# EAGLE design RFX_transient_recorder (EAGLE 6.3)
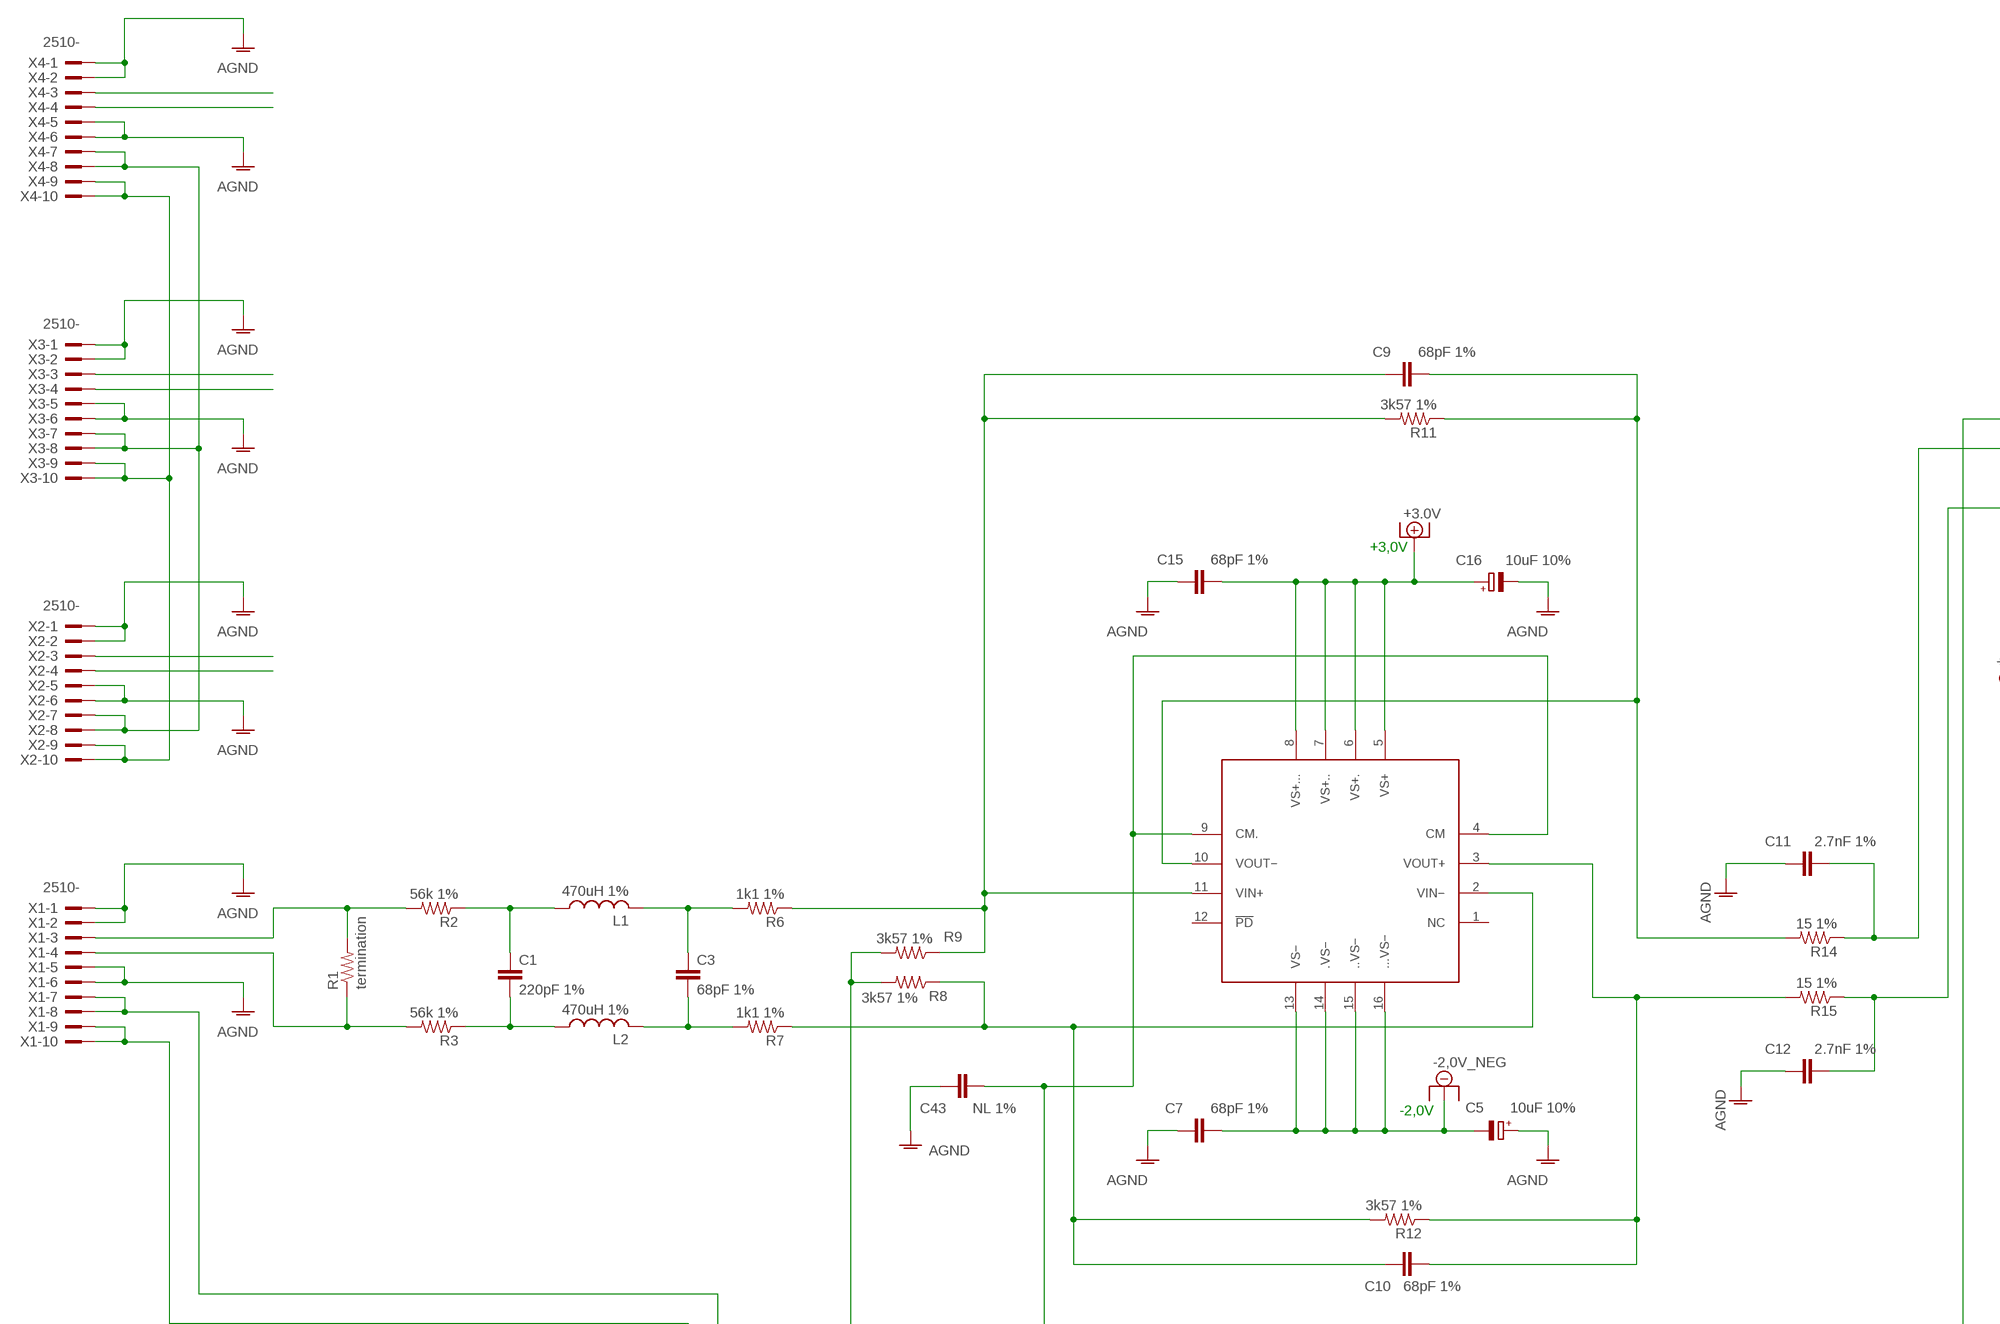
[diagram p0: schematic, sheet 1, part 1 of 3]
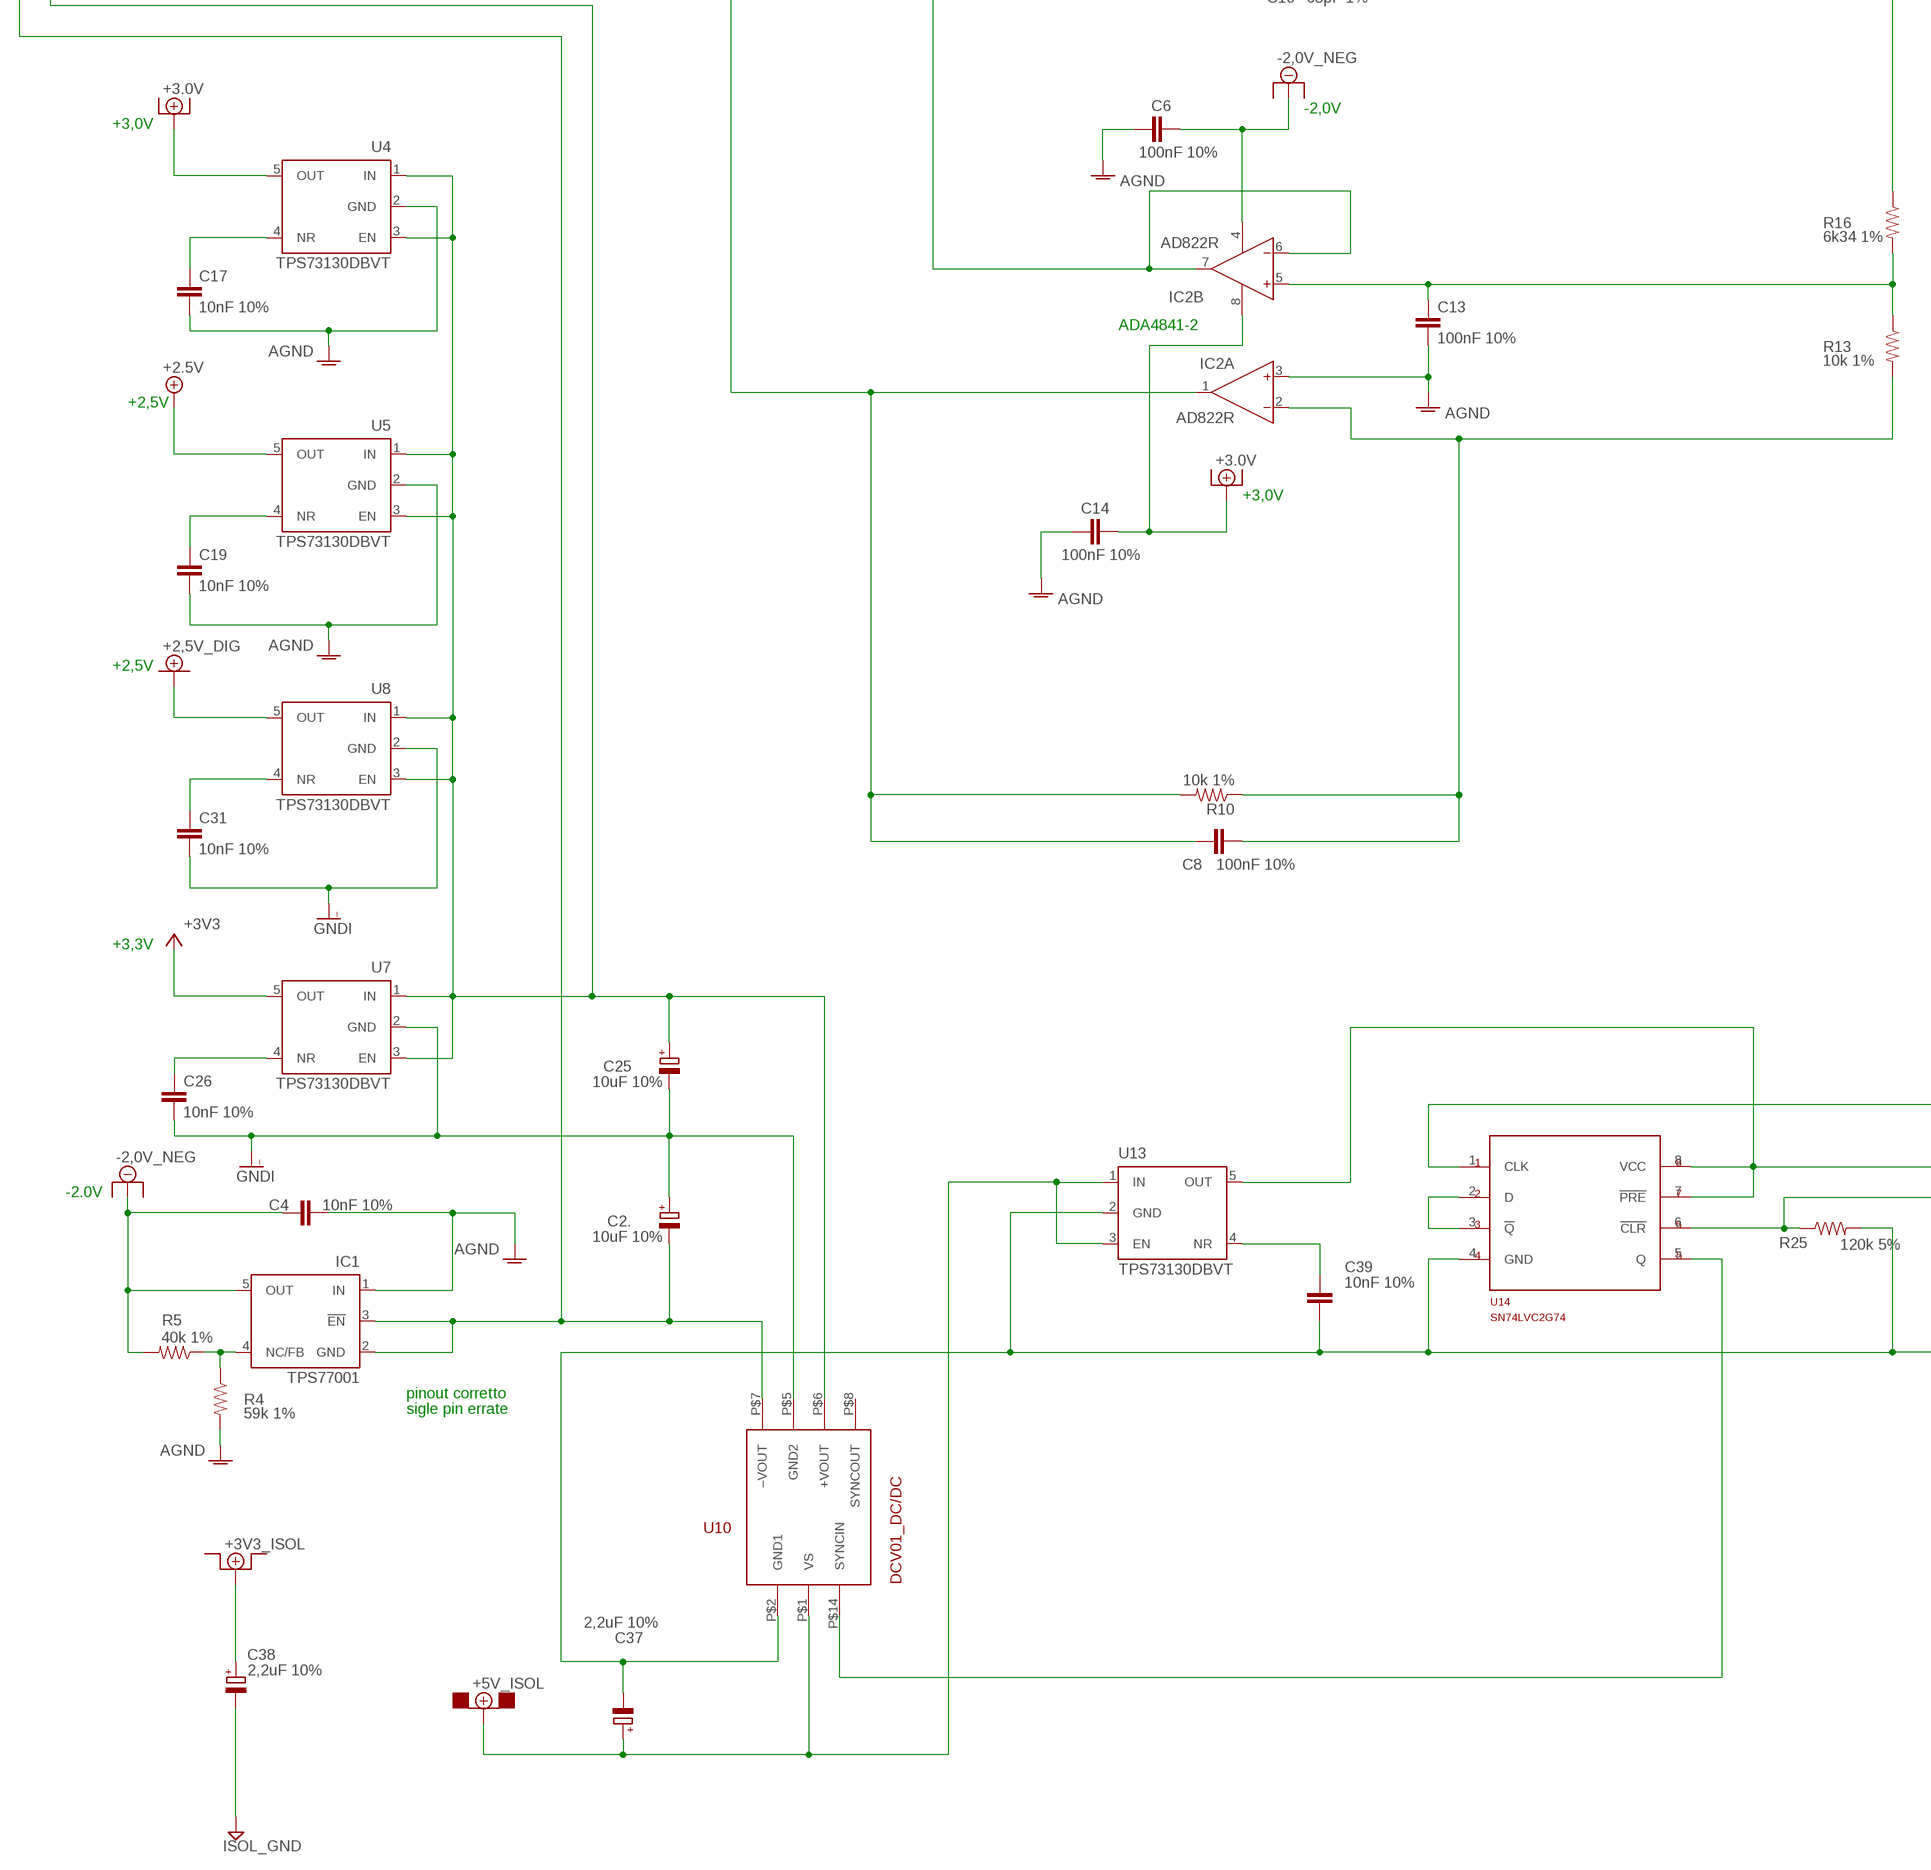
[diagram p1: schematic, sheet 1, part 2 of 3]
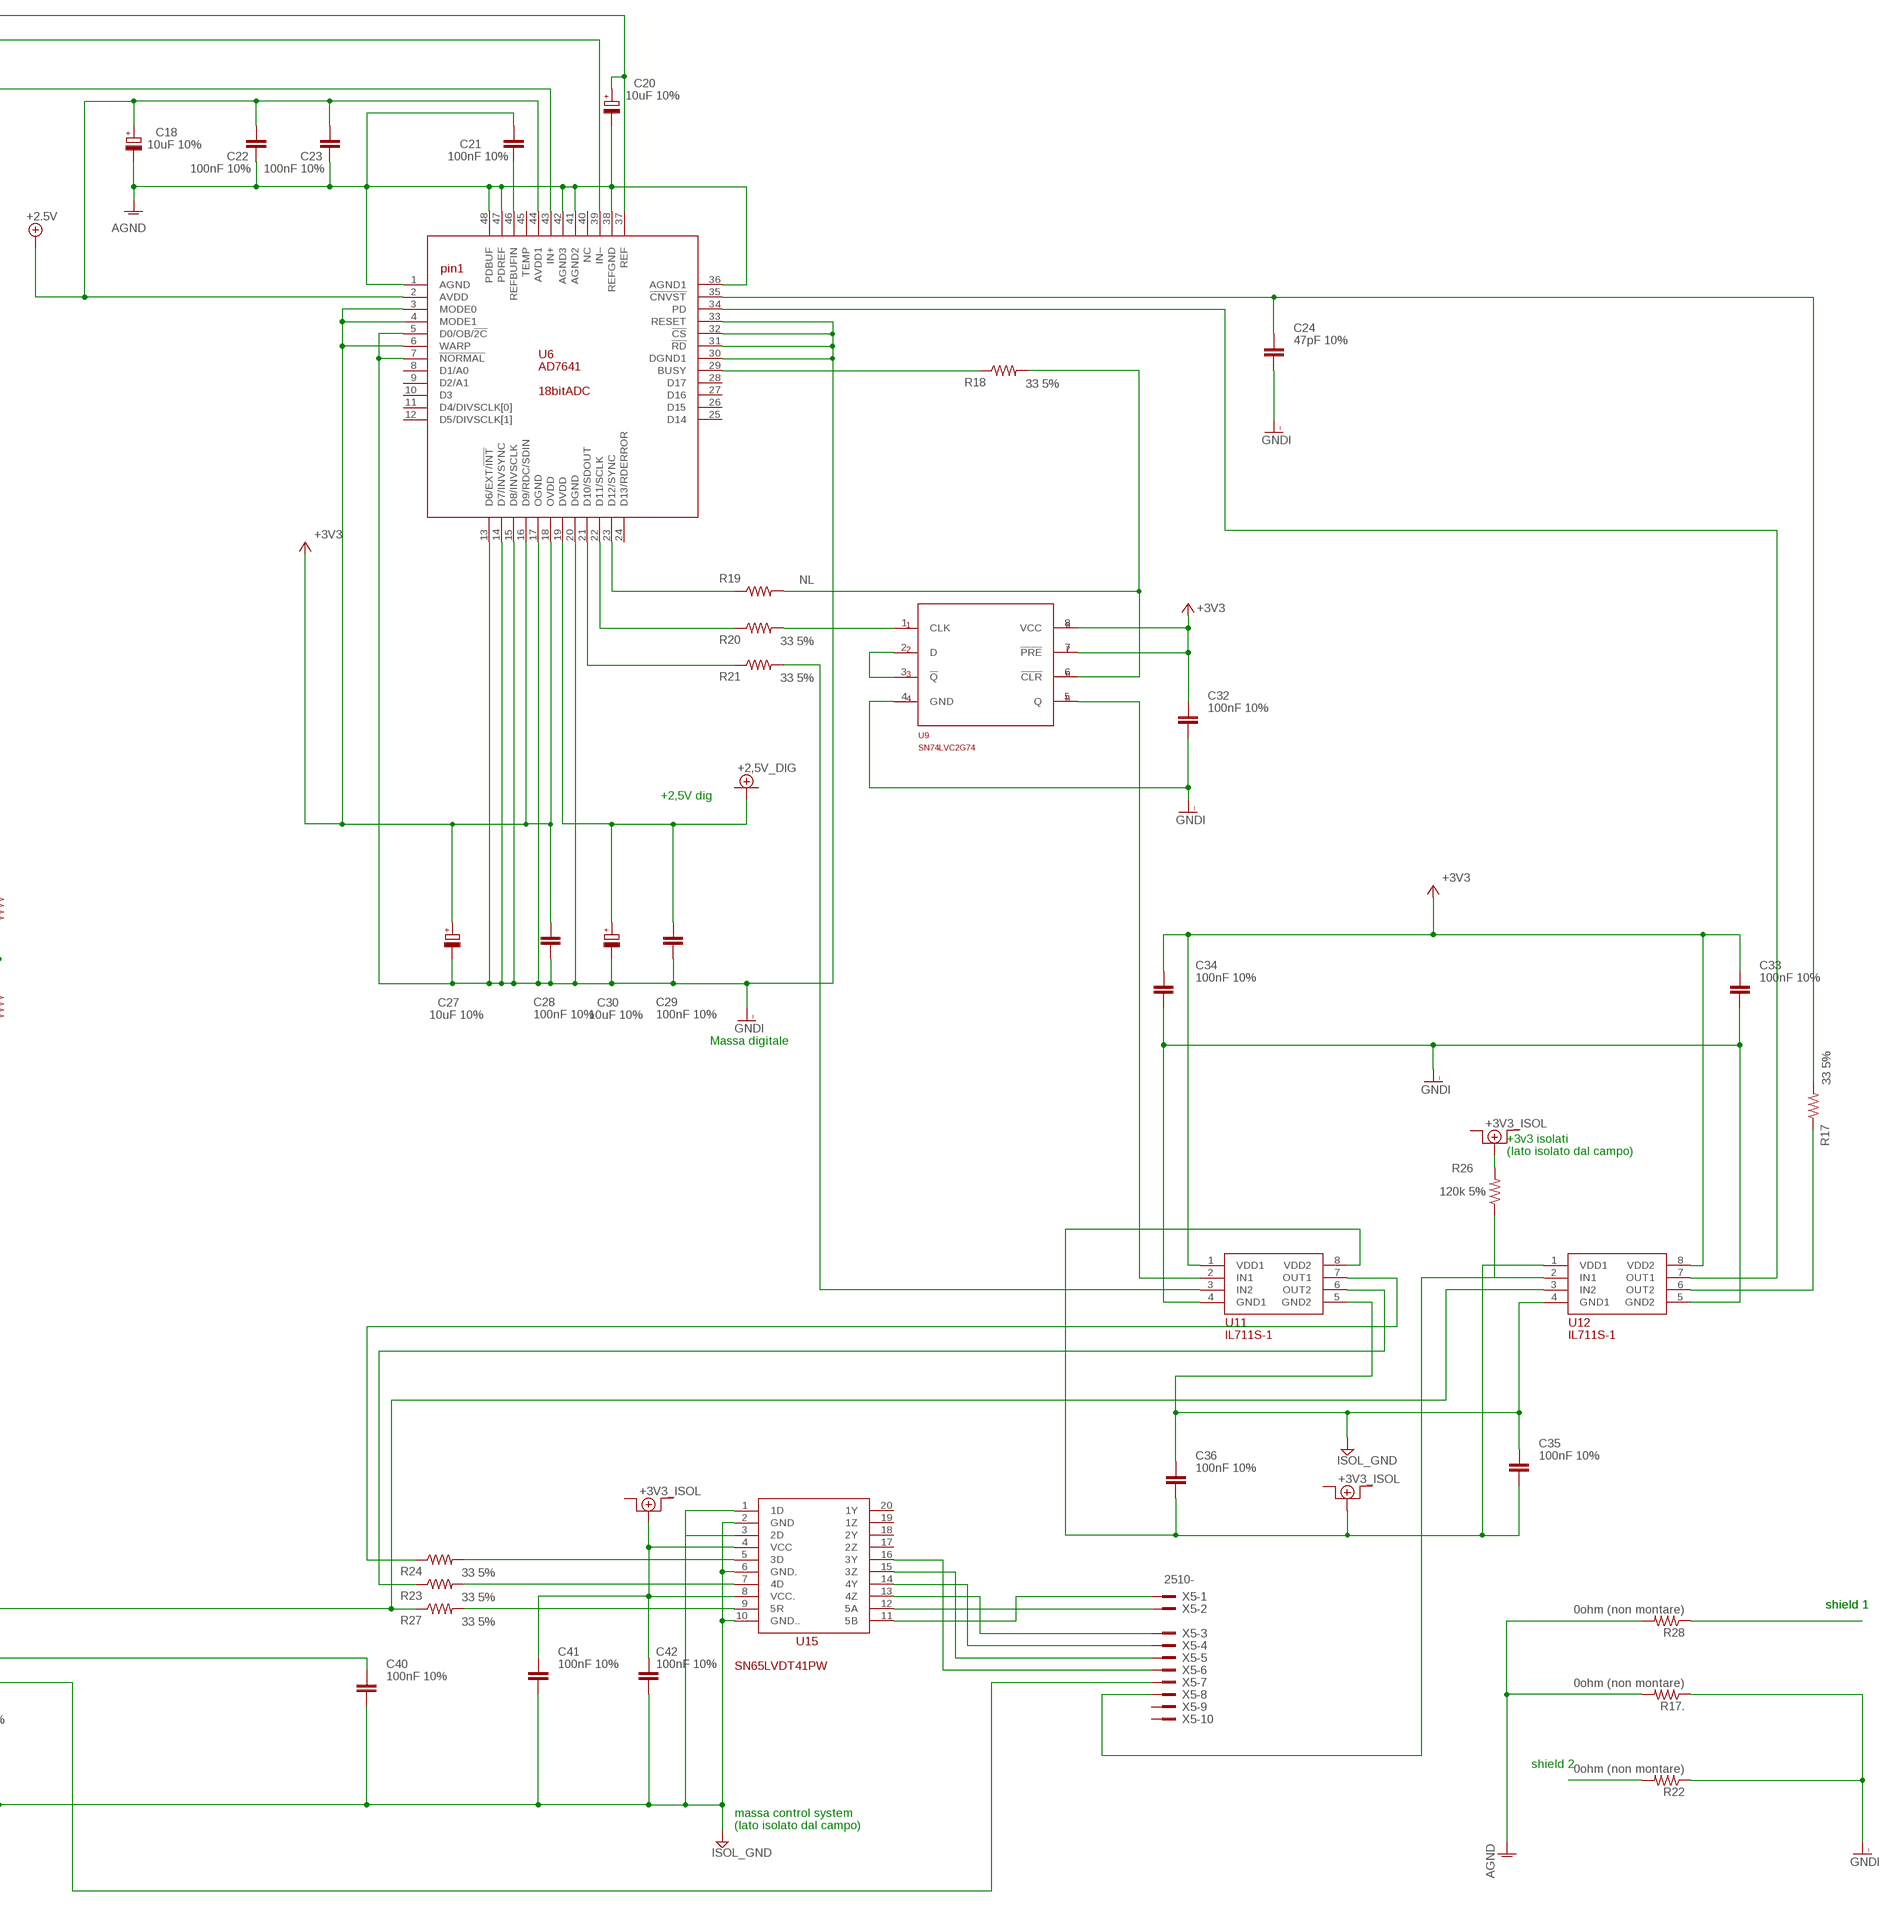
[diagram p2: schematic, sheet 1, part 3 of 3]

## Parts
C1  220pF 1%  C-EUC0402  [C0402]
C2.  10uF 10%  CPOL-EUSMCA  [SMC_A]
C3  68pF 1%  C-EUC0402  [C0402]
C4  10nF 10%  C-EUC0402  [C0402]
C5  10uF 10%  CPOL-EUSMCA  [SMC_A]
C6  100nF 10%  C-EUC0402  [C0402]
C7  68pF 1%  C-EUC0402  [C0402]
C8  100nF 10%  C-EUC0402  [C0402]
C9  68pF 1%  C-EUC0402  [C0402]
C10  68pF 1%  C-EUC0402  [C0402]
C11  2.7nF 1%  C-EUC0402  [C0402]
C12  2.7nF 1%  C-EUC0402  [C0402]
C13  100nF 10%  C-EUC0402  [C0402]
C14  100nF 10%  C-EUC0402  [C0402]
C15  68pF 1%  C-EUC0402  [C0402]
C16  10uF 10%  CPOL-EUSMCA  [SMC_A]
C17  10nF 10%  C-EUC0402  [C0402]
C18  10uF 10%  CPOL-EUSMCA  [SMC_A]
C19  10nF 10%  C-EUC0402  [C0402]
C20  10uF 10%  CPOL-EUSMCA  [SMC_A]
C21  100nF 10%  C-EUC0402  [C0402]
C22  100nF 10%  C-EUC0402  [C0402]
C23  100nF 10%  C-EUC0402  [C0402]
C24  47pF 10%  C-EUC0402  [C0402]
C25  10uF 10%  CPOL-EUSMCA  [SMC_A]
C26  10nF 10%  C-EUC0402  [C0402]
C27  10uF 10%  CPOL-EUSMCA  [SMC_A]
C28  100nF 10%  C-EUC0402  [C0402]
C29  100nF 10%  C-EUC0402  [C0402]
C30  10uF 10%  CPOL-EUSMCA  [SMC_A]
C31  10nF 10%  C-EUC0402  [C0402]
C32  100nF 10%  C-EUC0402  [C0402]
C33  100nF 10%  C-EUC0402  [C0402]
C34  100nF 10%  C-EUC0402  [C0402]
C35  100nF 10%  C-EUC0402  [C0402]
C36  100nF 10%  C-EUC0402  [C0402]
C37  2,2uF 10%  CPOL-EUSMCA  [SMC_A]
C38  2,2uF 10%  CPOL-EUSMCA  [SMC_A]
C39  10nF 10%  C-EUC0402  [C0402]
C40  100nF 10%  C-EUC0402  [C0402]
C41  100nF 10%  C-EUC0402  [C0402]
C42  100nF 10%  C-EUC0402  [C0402]
C43  NL 1%  C-EUC0402  [C0402]
IC1  TPS77001  [SOT23-DBV]
IC2  AD822R  [SO8]
L1  470uH 1%  L-USL3216C  [L3216C]
L2  470uH 1%  L-USL3216C  [L3216C]
R1  termination  R-US_R0402  [R0402]
R2  56k 1%  R-US_R0402  [R0402]
R3  56k 1%  R-US_R0402  [R0402]
R4  59k 1%  R-US_R0402  [R0402]
R5  40k 1%  R-US_R0402  [R0402]
R6  1k1 1%  R-US_R0402  [R0402]
R7  1k1 1%  R-US_R0402  [R0402]
R8  3k57 1%  R-US_R0402  [R0402]
R9  3k57 1%  R-US_R0402  [R0402]
R10  10k 1%  R-US_R0402  [R0402]
R11  3k57 1%  R-US_R0402  [R0402]
R12  3k57 1%  R-US_R0402  [R0402]
R13  10k 1%  R-US_R0402  [R0402]
R14  15 1%  R-US_R0402  [R0402]
R15  15 1%  R-US_R0402  [R0402]
R16  6k34 1%  R-US_R0402  [R0402]
R17  33 5%  R-US_R0402  [R0402]
R17.  0ohm (non montare)  R-US_R0402  [R0402]
R18  33 5%  R-US_R0402  [R0402]
R19  NL  R-US_R0402  [R0402]
R20  33 5%  R-US_R0402  [R0402]
R21  33 5%  R-US_R0402  [R0402]
R22  0ohm (non montare)  R-US_R0402  [R0402]
R23  33 5%  R-US_R0402  [R0402]
R24  33 5%  R-US_R0402  [R0402]
R25  120k 5%  R-US_R0402  [R0402]
R26  120k 5%  R-US_R0402  [R0402]
R27  33 5%  R-US_R0402  [R0402]
R28  0ohm (non montare)  R-US_R0402  [R0402]
U4  TPS73130DBVT  [SOT23-DBV]
U5  TPS73130DBVT  [SOT23-DBV]
U6  AD7641  [QFP-7X7-48]
U7  TPS73130DBVT  [SOT23-DBV]
U8  TPS73130DBVT  [SOT23-DBV]
U9  SN74LVC2G74  [SO-08]
U10  DCV01_DC/DCDCV010505DP_DC/DC_CONVERTER  [DCV10_DC/DC]
U11  IL711S-1  [SO-08]
U12  IL711S-1  [SO-08]
U13  TPS73130DBVT  [SOT23-DBV]
U14  SN74LVC2G74  [SO-08]
U15  SN65LVDT41PW  [TSSOP16]
U$1  THS4520_QFN16  [QFN16]
X1  2510-  [PAK100/2500-10]
X2  2510-  [PAK100/2500-10]
X3  2510-  [PAK100/2500-10]
X4  2510-  [PAK100/2500-10]
X5  2510-  [PAK100/2500-10]

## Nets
+2.5V: C18.+ C22.2 C23.2 U5.5(OUT) U6.2(AVDD) U6.44(AVDD1)
+2.5V_DIG: C29.2 C30.+ U6.19(DVDD) U8.5(OUT) ; supply symbol labelled +2,5V_DIG
+3.0V: C14.2 C15.2 C16.+ IC2.8(P:V+) U4.5(OUT) U$1.5(VS+) U$1.6(VS+.) U$1.7(VS+..) U$1.8(VS+...)
+3V3: C27.+ C28.2 C32.2 C33.2 C34.2 U6.3(MODE0) U6.4(MODE1) U6.6(WARP) U6.16(D9/RDC/SDIN) U6.18(OVDD) U7.5(OUT) U9.7(!PRE!) U9.8(VCC) U11.1(VDD1) U12.8(VDD2)
+3V3_ISOL: C35.1 C36.1 C38.+ C41.2 C42.2 R26.2 U11.8(VDD2) U12.1(VDD1) U15.4(VCC) U15.8(VCC.)
+5V_ISOL: C37.+ U10.P$1(VS) U13.1(IN) U13.3(EN)
-2.0V_NEG: C4.1 C5.- C6.2 C7.2 IC1.5(OUT) IC2.4(P:V-) R5.2 U$1.13(VS−) U$1.14(.VS−) U$1.15(..VS−) U$1.16(...VS−) ; supply symbol labelled -2,0V_NEG
AGND: C4.2 C5.+ C6.1 C7.1 C11.1 C12.1 C13.2 C14.1 C15.1 C16.- C17.2 C18.- C19.2 C20.- C21.2 C22.1 C23.1 C43.1 IC1.1(IN) IC2.3(A:IN+) R4.2 R17..2 R28.2 U4.2(GND) U5.2(GND) U6.1(AGND) U6.36(AGND1) U6.38(REFGND) U6.41(AGND2) U6.42(AGND3) U6.47(PDREF) U6.48(PDBUF) X1.1 X1.2 X1.5 X1.6 X2.1 X2.2 X2.5 X2.6 X3.1 X3.2 X3.5 X3.6 X4.1 X4.2 X4.5 X4.6
GNDI: C2..+ C24.1 C25.- C26.2 C27.- C28.1 C29.1 C30.- C31.2 C32.1 C33.1 C34.1 R17..1 R22.1 U6.5(D0/OB/!2C!) U6.7(!NORMAL!) U6.13(D6/EXT/!INT!) U6.14(D7/INVSYNC) U6.15(D8/INVSCLK) U6.17(OGND) U6.20(DGND) U6.30(DGND1) U6.31(!RD!) U6.32(!CS!) U6.33(RESET) U7.2(GND) U8.2(GND) U9.4(GND) U10.P$5(GND2) U11.4(GND1) U12.5(GND2)
ISOL_GND: C35.2 C36.2 C37.- C38.- C39.1 C40.1 C41.1 C42.1 R25.2 U10.P$2(GND1) U11.5(GND2) U12.4(GND1) U13.2(GND) U14.4(GND) U15.1(1D) U15.2(GND) U15.3(2D) U15.6(GND.) U15.10(GND..)
N$1: C3.1 L1.2 R6.2
N$2: C1.1 L1.1 R2.1
N$3: C3.2 L2.2 R7.2
N$4: C1.2 L2.1 R3.1
N$5: C9.1 R6.1 R9.1 R11.2 U$1.11(VIN+)
N$6: C10.1 R7.1 R8.1 R12.2 U$1.2(VIN−)
N$7: R20.2 U9.1(CLK)
N$8: R1.2 R2.2 X1.3
N$9: R1.1 R3.2 X1.4
N$10: C9.2 R11.1 R14.2 U$1.10(VOUT−)
N$11: C10.2 R12.1 R15.2 U$1.3(VOUT+)
N$12: C11.2 R14.1 U6.39(IN–)
N$13: C12.2 R15.1 U6.43(IN+)
N$14: R28.1
N$15: R22.2
N$16: C2..- IC1.2(GND) IC1.3(!EN) U10.P$7(–VOUT) X1.9 X1.10
N$17: C17.1 U4.4(NR)
N$18: C25.+ U4.1(IN) U4.3(EN) U5.1(IN) U5.3(EN) U7.1(IN) U7.3(EN) U8.1(IN) U8.3(EN) U10.P$6(+VOUT) X1.7 X1.8
N$19: X2.3
N$20: C19.1 U5.4(NR)
N$21: X2.4
N$22: X2.9 X2.10 X3.9 X3.10 X4.9 X4.10
N$23: C31.1 U8.4(NR)
N$24: X2.7 X2.8 X3.7 X3.8 X4.7 X4.8
N$25: X3.3
N$26: C26.1 U7.4(NR)
N$27: IC1.4(NC/FB) R4.1 R5.1
N$28: C43.2 IC2.6(B:IN-) IC2.7(B:OUT) U$1.4(CM) U$1.9(CM.)
N$29: X3.4
N$30: C13.1 IC2.5(B:IN+) R13.1 R16.2
N$31: R20.1 U6.22(D11/SCLK)
N$32: C20.+ R16.1 U6.37(REF)
N$33: C21.1 U6.46(REFBUFIN)
N$34: U15.11(5B) X5.1
N$35: U15.12(5A) X5.2
N$36: R19.1 U6.23(D12/SYNC)
N$37: R18.2 R19.2 U9.6(!CLR!)
N$38: R18.1 U6.29(BUSY)
N$39: U9.2(D) U9.3(!Q!)
N$40: C8.1 IC2.1(A:OUT) R8.2 R9.2 R10.2
N$41: C8.2 IC2.2(A:IN-) R10.1 R13.2
N$42: U9.5(Q) U11.2(IN1)
N$43: R21.1 U6.21(D10/SDOUT)
N$44: R21.2 U11.3(IN2)
N$45: C24.2 R17.2 U6.35(!CNVST!)
N$46: R17.1 U12.6(OUT2)
N$47: U6.34(PD) U12.7(OUT1)
N$48: X4.3
N$49: X4.4
N$50: R27.1 U12.3(IN2) U14.1(CLK)
N$51: R24.2 U15.5(3D)
N$52: R23.2 U15.7(4D)
N$53: R24.1 U11.7(OUT1)
N$54: R23.1 U11.6(OUT2)
N$55: U15.13(4Z) X5.3
N$56: R27.2 U15.9(5R)
N$57: R26.1 U12.2(IN1) X5.8
N$58: U15.14(4Y) X5.4
N$59: U14.2(D) U14.3(!Q!)
N$60: R25.1 U14.6(!CLR!) X5.7
N$61: U10.P$14(SYNCIN) U14.5(Q)
N$62: C40.2 U13.5(OUT) U14.7(!PRE!) U14.8(VCC)
N$63: U15.15(3Z) X5.5
N$64: C39.2 U13.4(NR)
N$65: U15.16(3Y) X5.6
Unconnected: U6.8(D1/A0) U6.9(D2/A1) U6.10(D3) U6.11(D4/DIVSCLK[0]) U6.12(D5/DIVSCLK[1]) U6.24(D13/RDERROR) U6.25(D14) U6.26(D15) U6.27(D16) U6.28(D17) U6.40(NC) U6.45(TEMP) U10.P$8(SYNCOUT) U15.17(2Z) U15.18(2Y) U15.19(1Z) U15.20(1Y) U$1.1(NC) U$1.12(!PD!) X5.9 X5.10

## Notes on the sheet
- +3,0V
- -2,0V
- +2,5V dig
- -2,0V
- +3,0V
- ADA4841-2
- Massa digitale
- +2,5V
- +3,0V
- +3v3 isolati
- (lato isolato dal campo)
- +2,5V
- +3,3V
- shield 1 | shield 1
- -2.0V
- shield 2
- massa control system
- (lato isolato dal campo)
- pinout corretto
- sigle pin errate

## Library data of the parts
C1 C3 C4 C6-C15 C17 C19 C21-C24 C26 C28 C29 C31-C36 C39-C43 = resistor:C-EU: CAPACITOR, European symbol
C2. C5 C16 C18 C20 C25 C27 C30 C37 C38 = resistor:CPOL-EU: POLARIZED CAPACITOR, European symbol
IC1 = texas:TPS770*: ULTRALOW-POWER 50-mA LOW-DROPOUT LINEAR REGULATORS 50-mA Low-Dropout Regulator Source: http://focus.ti.com/lit/ds/symlink/tps77001.pdf; MF: TEXAS INSTRUMENTS; MPN: TPS77001DBVT; OC_FARNELL: 8461554; OC_NEWARK: 77C1171
IC2 = analog-devices:AD822: Single-Supply, Rail-to-Rail Low Power FET-Input Op Amp Source: http://www.analog.com/static/imported-files/data_sheets/AD822.pdf; MF: ANALOG DEVICES; MPN: AD822BRZ; OC_FARNELL: 1651303
L1 L2 = resistor:L-US: INDUCTOR, American symbol
R1-R17 R17. R18-R28 = resistor:R-US_: RESISTOR, American symbol
U4 U5 U7 U8 U13 = TPS73130DBVT:TPS73130DBVT
U6 = AD7641:AD7641
U9 U14 = SN74LVC2G74DCUR_SOP8:SN74LVC2G74
U10 = DCV01_DCDC:DCV01_DC/DC
U11 U12 = IL711S-1 SOIC8:IL711S-1
U15 = SN65LVDT41PW-TSSOP20:SN65LVDT41PW: MEMORY STICK™ INTERCONNECT EXTENDER CHIPSET WITH LVDS
U$1 = THS4520 QFN16:THS4520_QFN16
X1-X5 = con-3m:2510-: 3M (TM) Pak 100 4-Wall Header Source: 3M; MF: 3M; MPN: 2510-6002UB; OC_FARNELL: 9838244; OC_NEWARK: 46F4725

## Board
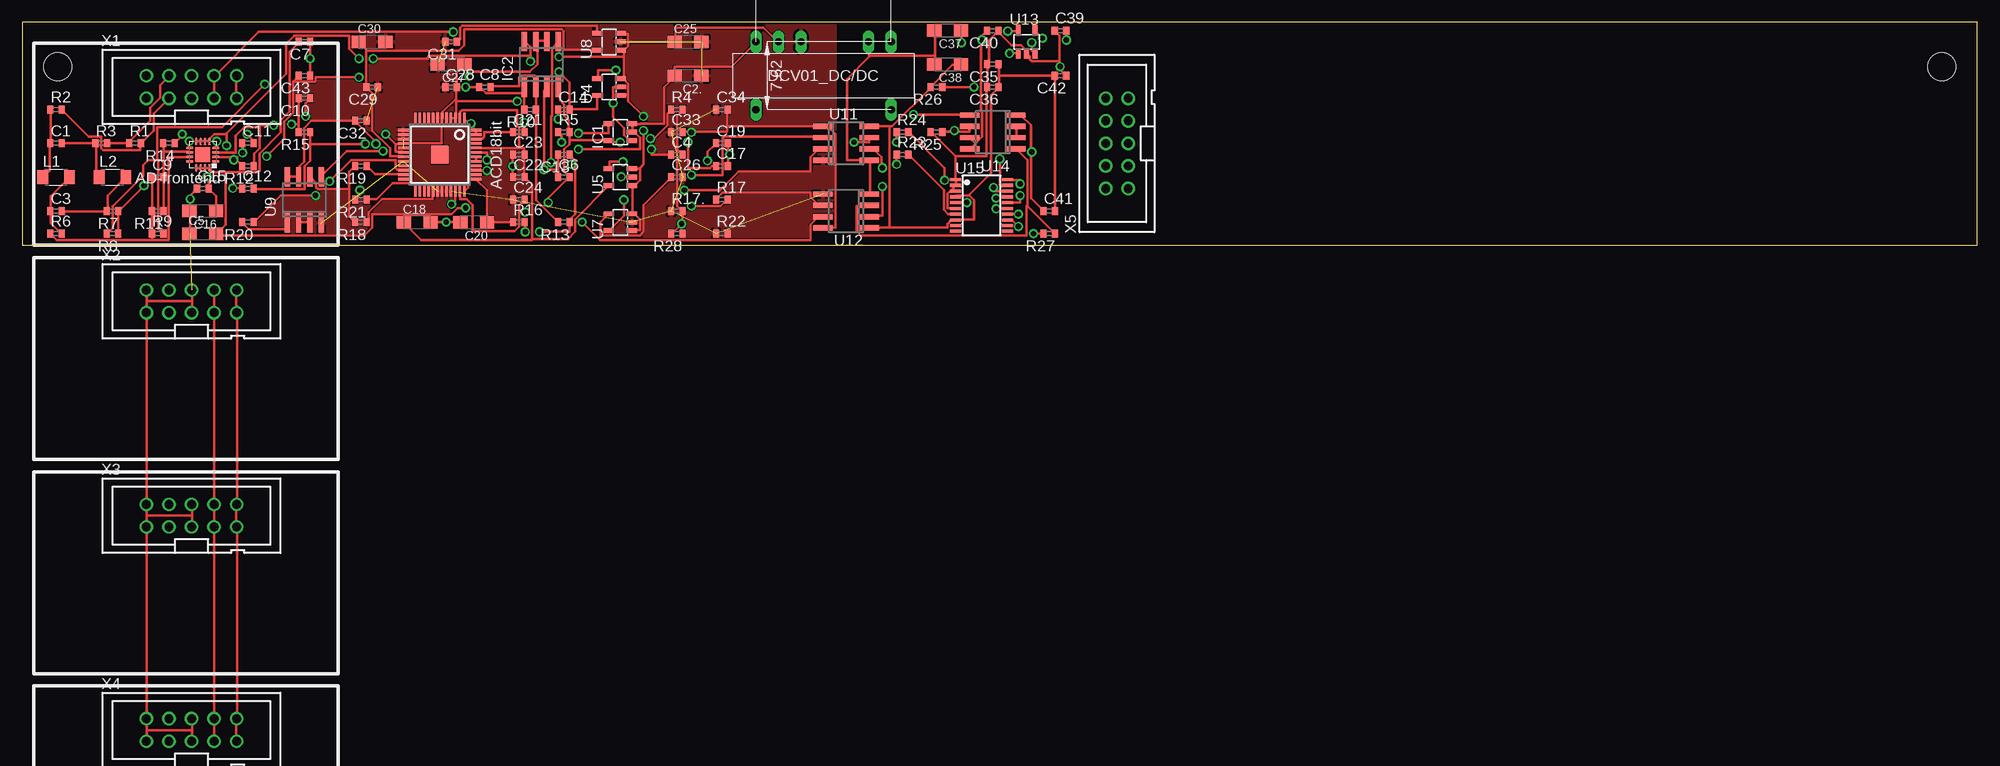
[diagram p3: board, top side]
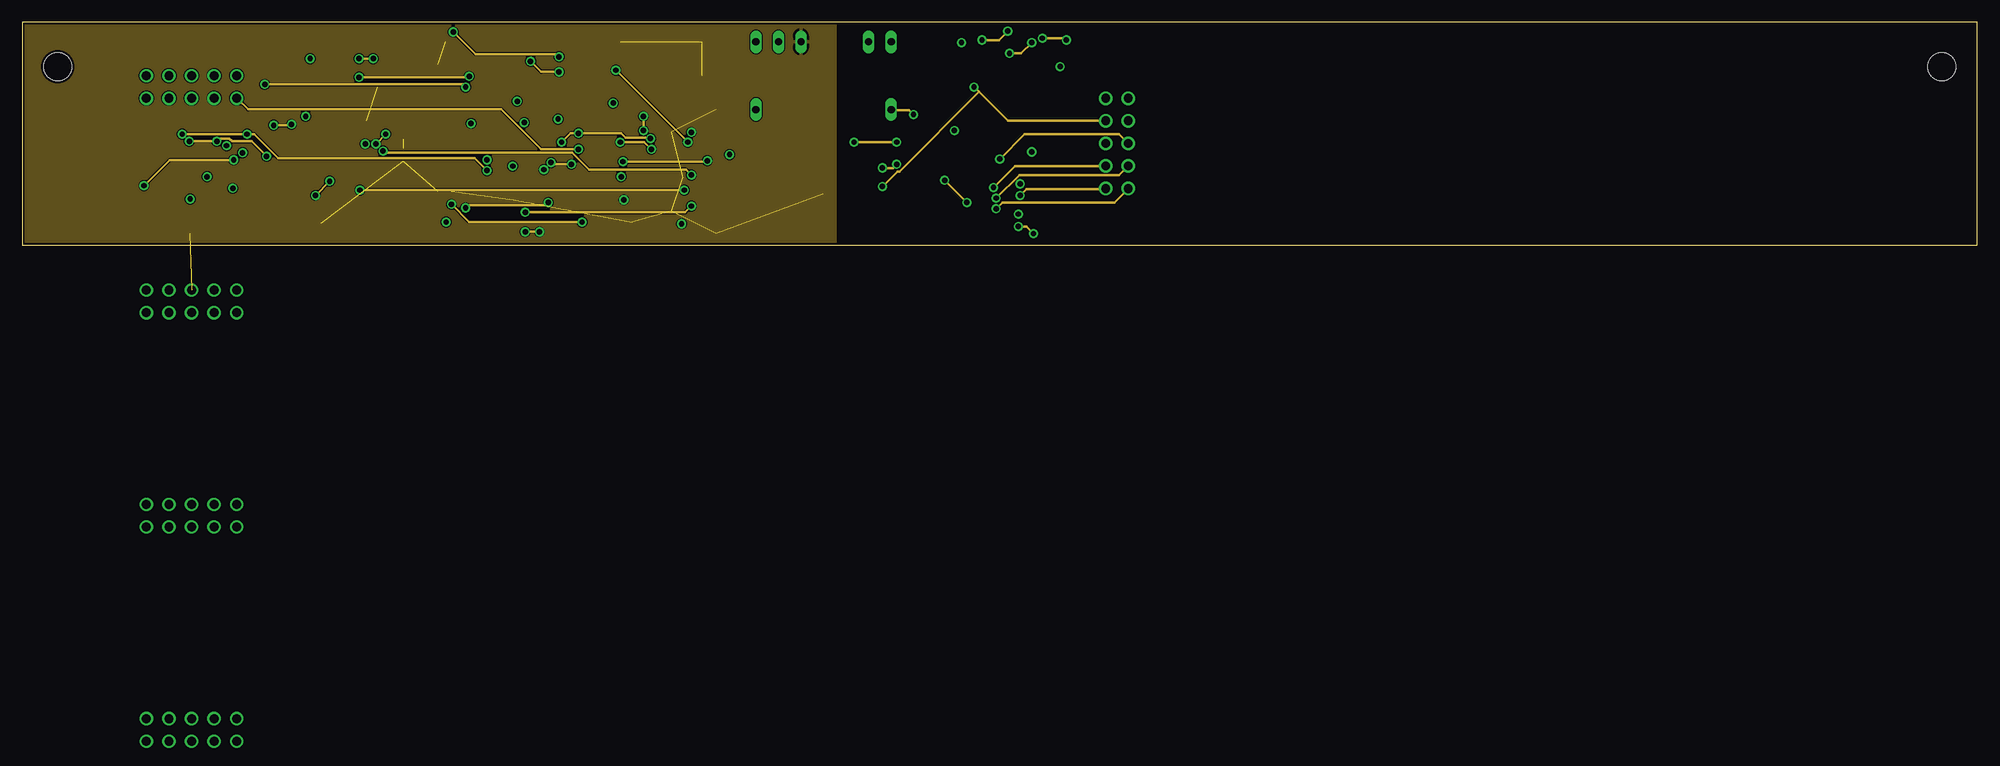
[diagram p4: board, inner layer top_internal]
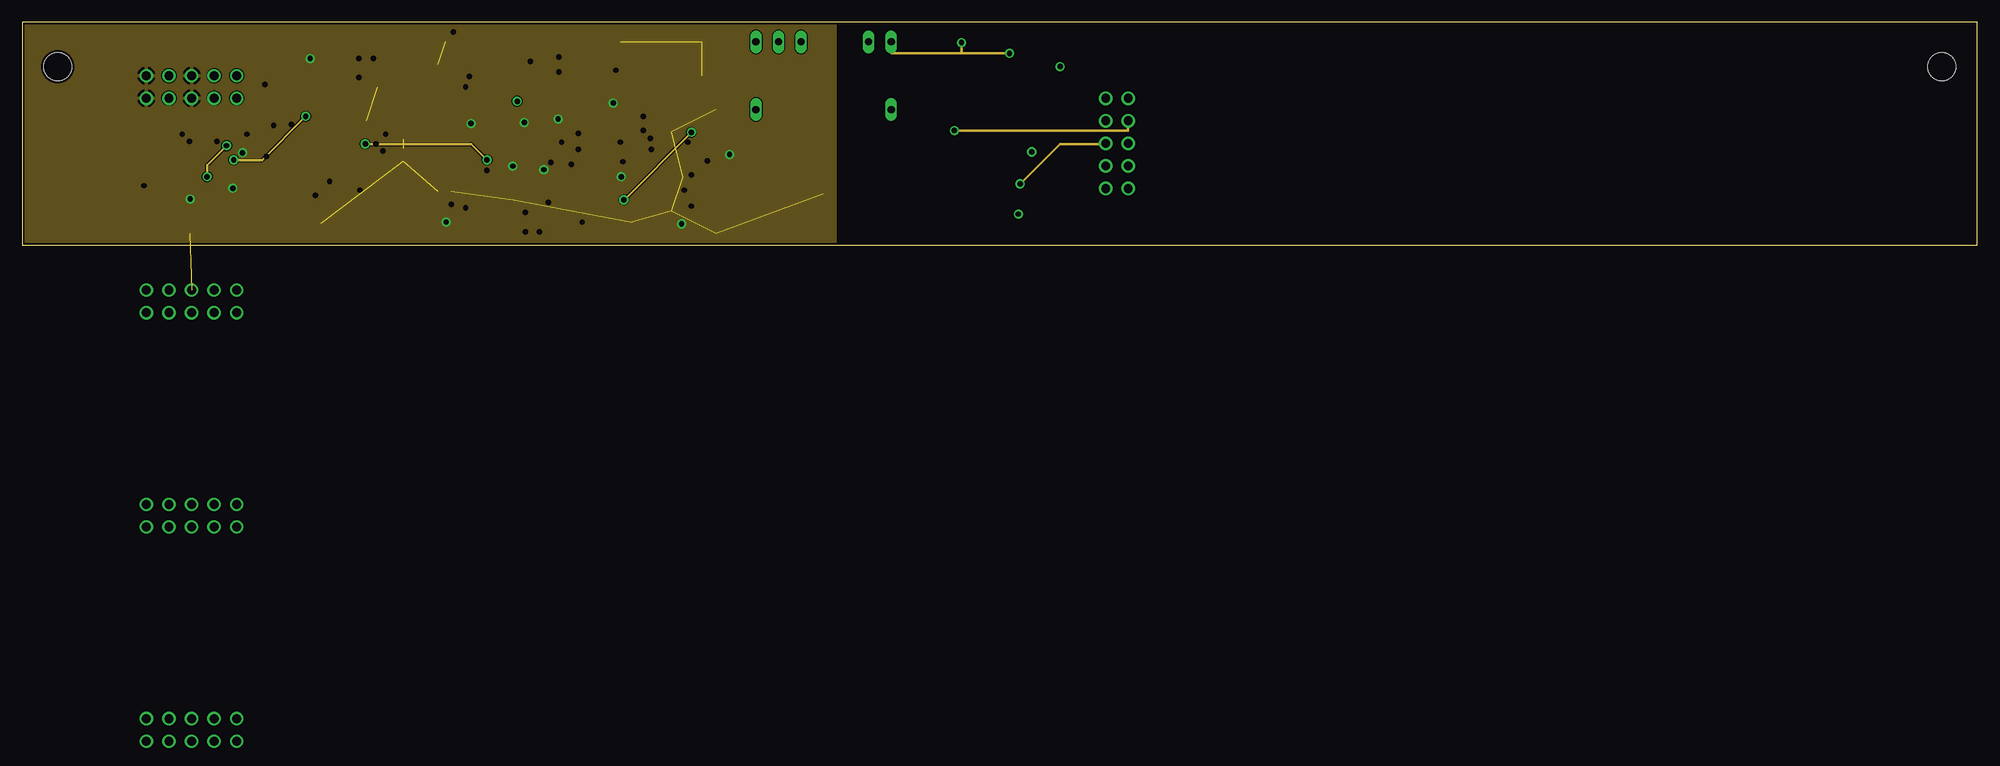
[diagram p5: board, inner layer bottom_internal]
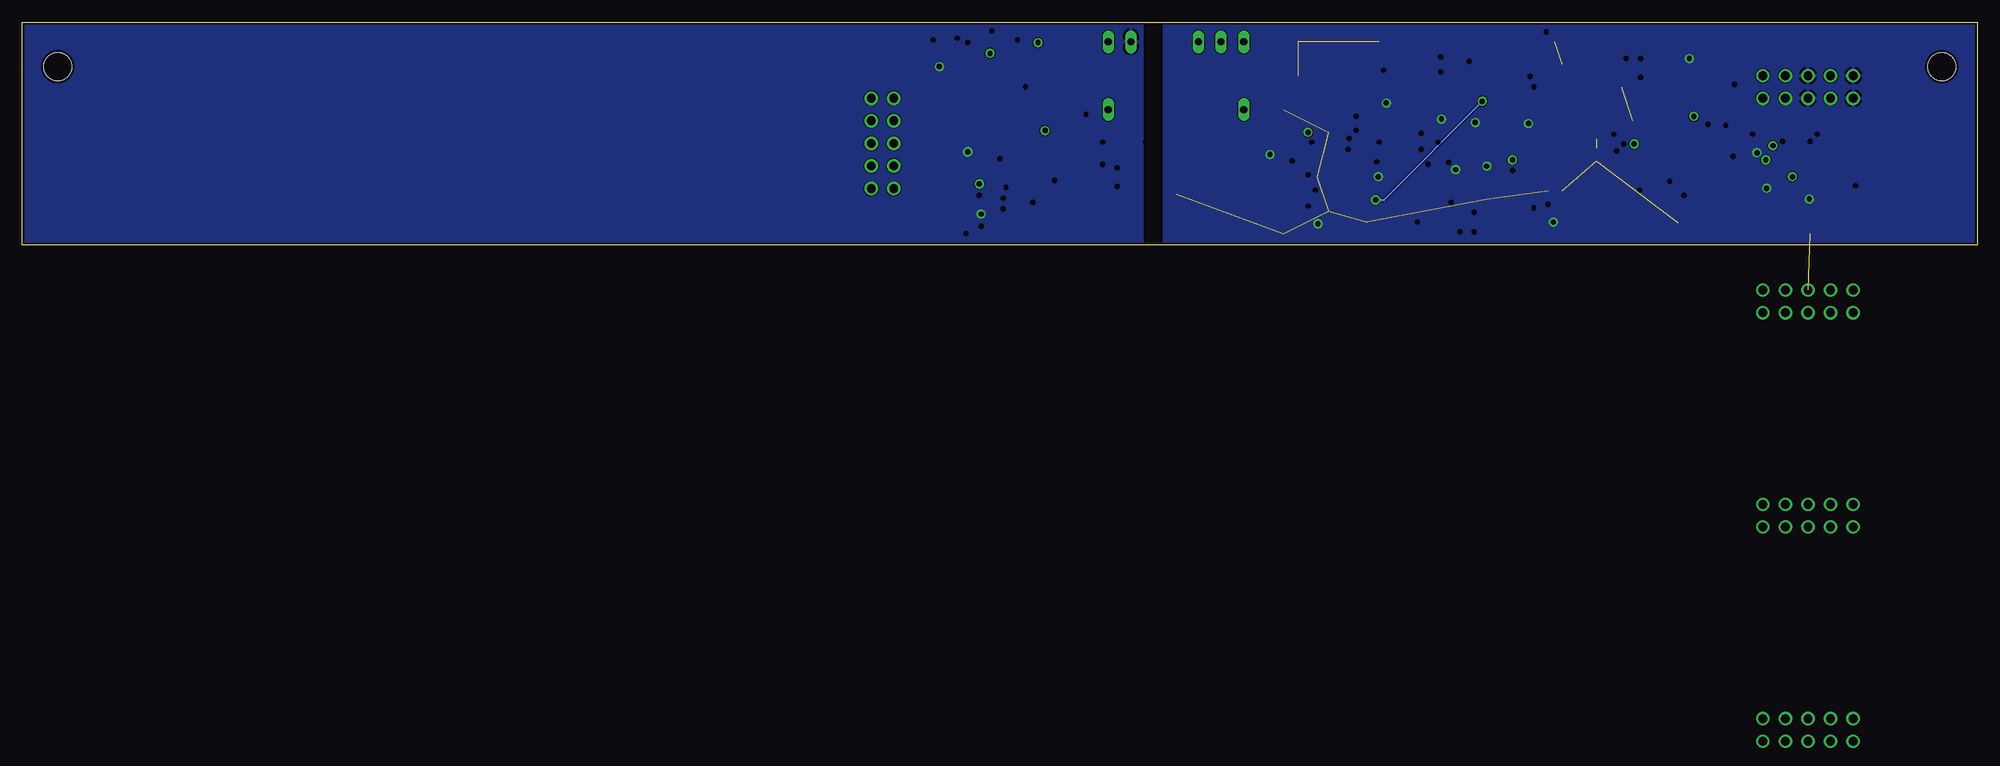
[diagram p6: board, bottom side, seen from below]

Size 220 x 25.07 mm. Coordinates in mm from the lower left corner, seen from the top.
Outline: 0,0 220,0 220,25.07 0,25.07 0,0
Copper layers ((1*2)+(15*16)): Top 0.035mm / dielectric 1.5mm / top_internal 0.035mm / dielectric 0.15mm / bottom_internal 0.035mm / dielectric 0.2mm / Bottom 0.035mm
Design rules "default *": minimum track width 10mil, minimum drill 24mil, track to track 4mil, track to pad 4mil, pad to pad 4mil, via to via 4mil, smd to smd 1mil, copper to edge 10mil, drill to drill 8mil, minimum pad ring 10mil, minimum via ring 8mil, stop-mask expansion 4mil, vias tented up to drill 0mil, thermal gap 10mil
Holes 3.2 mm at 4,20.07 4,-69.93 216,20.07 216,-69.93

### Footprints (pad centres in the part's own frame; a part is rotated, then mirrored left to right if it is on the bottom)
C0402 = smd 0.7 x 0.9: 1 -0.65,0; 2 0.65,0
SMC_A = smd 1.6 x 1.4: + -1.5,0; - 1.5,0
SOT23-DBV = smd 0.55 x 1.2: 1 -0.95,-1.3; 2 0,-1.3; 3 0.95,-1.3; 4 0.95,1.3; 5 -0.95,1.3
SO8 = smd 0.6 x 2.2: 1 -1.905,-2.6; 2 -0.635,-2.6; 3 0.635,-2.6; 4 1.905,-2.6; 5 1.905,2.6; 6 0.635,2.6; 7 -0.635,2.6; 8 -1.905,2.6
L3216C = smd 1.2 x 1.6: 1 -1.5,0; 2 1.5,0
R0402 = smd 0.7 x 0.9: 1 -0.65,0; 2 0.65,0
QFP-7X7-48 = smd 0.3 x 1.2: 1 -2.75,-4.1; 2 -2.25,-4.1; 3 -1.75,-4.1; 4 -1.25,-4.1; 5 -0.75,-4.1; 6 -0.25,-4.1; 7 0.25,-4.1; 8 0.75,-4.1; 9 1.25,-4.1; 10 1.75,-4.1; 11 2.25,-4.1; 12 2.75,-4.1; 25 2.75,4.1; 26 2.25,4.1; 27 1.75,4.1; 28 1.25,4.1; 29 0.75,4.1; 30 0.25,4.1; 31 -0.25,4.1; 32 -0.75,4.1; 33 -1.25,4.1; 34 -1.75,4.1; 35 -2.25,4.1; 36 -2.75,4.1 | smd 1.2 x 0.3: 13 4.1,-2.75; 14 4.1,-2.25; 15 4.1,-1.75; 16 4.1,-1.25; 17 4.1,-0.75; 18 4.1,-0.25; 19 4.1,0.25; 20 4.1,0.75; 21 4.1,1.25; 22 4.1,1.75; 23 4.1,2.25; 24 4.1,2.75; 37 -4.1,2.75; 38 -4.1,2.25; 39 -4.1,1.75; 40 -4.1,1.25; 41 -4.1,0.75; 42 -4.1,0.25; 43 -4.1,-0.25; 44 -4.1,-0.75; 45 -4.1,-1.25; 46 -4.1,-1.75; 47 -4.1,-2.25; 48 -4.1,-2.75 | smd 2 x 2: EXP 0,0
SO-08 = smd 0.6 x 2.2: 1 -1.905,-2.6; 2 -0.635,-2.6; 3 0.635,-2.6; 4 1.905,-2.6; 5 1.905,2.6; 6 0.635,2.6; 7 -0.635,2.6; 8 -1.905,2.6
DCV10_DC/DC = drill 0.8 long: P$1 -3.81,8.89; P$2 -3.81,6.35; P$5 -3.81,-1.27; P$6 -3.81,-3.81; P$7 -3.81,-6.35; P$8 3.81,-6.35; P$14 3.81,8.89
TSSOP16 = smd 0.35 x 1.2: 1 -2.275,-2.925; 2 -1.625,-2.925; 3 -0.975,-2.925; 4 -0.325,-2.925; 5 0.325,-2.925; 6 0.975,-2.925; 7 1.625,-2.925; 8 2.275,-2.925; 9 2.275,2.925; 10 1.625,2.925; 11 0.975,2.925; 12 0.325,2.925; 13 -0.325,2.925; 14 -0.975,2.925; 15 -1.625,2.925; 16 -2.275,2.925; 17 2.895,-2.925; 18 3.545,-2.925; 19 3.545,2.925; 20 2.895,2.925
QFN16 = smd 0.85 x 0.3: 1 -1.475,0.75; 2 -1.475,0.25; 3 -1.475,-0.25; 4 -1.475,-0.75; 9 1.475,-0.75; 10 1.475,-0.25; 11 1.475,0.25; 12 1.475,0.75 | smd 0.3 x 0.85: 5 -0.75,-1.475; 6 -0.25,-1.475; 7 0.25,-1.475; 8 0.75,-1.475; 13 0.75,1.475; 14 0.25,1.475; 15 -0.25,1.475; 16 -0.75,1.475 | smd 1.7 x 1.7: TH 0,0
PAK100/2500-10 = drill 1 pad 1.422: 1 -5.08,-1.27; 2 -5.08,1.27; 3 -2.54,-1.27; 4 -2.54,1.27; 5 0,-1.27; 6 0,1.27; 7 2.54,-1.27; 8 2.54,1.27; 9 5.08,-1.27; 10 5.08,1.27

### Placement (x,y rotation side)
C1  3.81,11.43 0 top
C2.  74.93,19.05 180 top
C3  3.81,3.81 0 top
C4  73.66,10.16 0 top
C5  20.32,1.27 0 top
C6  60.96,7.62 0 top
C7  31.75,22.86 180 top
C8  52.07,17.78 0 top
C9  15.24,7.62 0 top
C10  31.75,16.51 180 top
C11  25.4,11.43 0 top
C12  25.4,6.35 0 top
C13  60.96,10.16 180 top
C14  60.96,15.24 0 top
C15  20.32,6.35 0 top
C16  20.32,3.81 180 top
C17  78.74,8.89 0 top
C18  44.45,2.54 0 top
C19  78.74,11.43 0 top
C20  50.8,2.54 180 top
C21  55.88,12.7 0 top
C22  55.88,7.62 0 top
C23  55.88,10.16 0 top
C24  55.88,5.08 0 top
C25  74.93,22.86 0 top
C26  73.66,7.62 0 top
C27  48.26,20.32 180 top
C28  48.26,17.78 0 top
C29  39.37,17.78 180 top
C30  39.37,22.86 0 top
C31  48.26,22.86 180 top
C32  38.1,13.97 180 top
C33  73.66,12.7 0 top
C34  78.74,15.24 0 top
C35  109.22,20.32 180 top
C36  109.22,17.78 180 top
C37  104.14,24.13 180 top
C38  104.14,20.32 180 top
C39  116.84,24.13 0 top
C40  109.22,24.13 180 top
C41  115.57,3.81 0 top
C42  116.84,19.05 180 top
C43  31.75,19.05 180 top
IC1  67.31,12.7 90 top
IC2  58.42,20.32 0 top
L1  3.81,7.62 0 top
L2  10.16,7.62 0 top
R1  12.7,11.43 0 top
R2  3.81,15.24 0 top
R3  8.89,11.43 0 top
R4  73.66,15.24 0 top
R5  60.96,12.7 0 top
R6  3.81,1.27 0 top
R7  10.16,3.81 180 top
R8  10.16,1.27 180 top
R9  15.24,1.27 0 top
R10  57.15,15.24 180 top
R11  15.24,3.81 180 top
R12  25.4,8.89 180 top
R13  60.96,2.54 180 top
R14  16.51,11.43 180 top
R15  31.75,12.7 180 top
R16  55.88,2.54 0 top
R17  78.74,5.08 0 top
R17.  73.66,3.81 0 top
R18  38.1,2.54 180 top
R19  38.1,8.89 180 top
R20  25.4,2.54 180 top
R21  38.1,5.08 180 top
R22  78.74,1.27 0 top
R23  99.06,10.16 0 top
R24  99.06,12.7 0 top
R25  102.87,12.7 180 top
R26  102.87,17.78 180 top
R27  115.57,1.27 180 top
R28  73.66,1.27 180 top
U4  66.04,17.78 90 top
U5  67.31,7.62 90 top
U6  46.99,10.16 180 top
U7  67.31,2.54 90 top
U8  66.04,22.86 90 top
U9  31.75,5.08 0 top
U10  88.9,19.05 270 top
U11  92.71,11.43 270 top
U12  92.71,3.81 90 top
U13  113.03,22.86 0 top
U14  109.22,12.7 90 top
U15  107.95,5.08 270 top
U$1  20.32,10.16 180 top
X1  19.05,17.78 0 top
X2  19.05,-6.35 0 top  (outside the outline)
X3  19.05,-30.48 0 top  (outside the outline)
X4  19.05,-54.61 0 top  (outside the outline)
X5  123.19,11.43 90 top

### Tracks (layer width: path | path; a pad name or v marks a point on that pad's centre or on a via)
+2.5V
  Top 0.254: 55.9,10.87 56.5,10.87 56.5,10.27 C23.2 56.5,10.07 56.5,7.67 C22.2 56.6,7.57 57.4,6.77 57.4,0.67 | 55.9,10.87 51.1,10.87 U6.44 | 55.9,10.87 55.9,13.17 55.7,13.37 55.7,15.17 49.5,15.17 49.3,14.97 49.3,14.27 U6.2 | 57.4,0.67 61.4,0.67 62.2,1.47 62.2,2.87 U5.5 | C18.+ 43,2.47 44.9,0.57 57.3,0.57 57.3,0.67 57.4,0.67
+2.5V_DIG
  Top 0.254: 38.7,21.87 38.7,21.97 37.9,22.77 C30.+ | 38.7,21.87 38.7,17.87 C29.2 38.8,17.67 39.4,17.07 39.4,12.87 41.4,10.87 41.4,9.97 42.8,9.97 U6.19 | 38.7,21.87 49.1,21.87 49.7,22.47 49.7,24.27 60.7,24.27 60.9,24.07 60.9,21.97 64.7,21.97 U8.5
+3.0V  (via drill 0.61, 0.61 layers 1-2)
  Top 0.254: U$1.8 19.6,11.67 20,11.67 U$1.7 20.1,11.67 20.5,11.67 U$1.6 20.6,11.67 21,11.67 U$1.5 21,11.77 21.1,11.87 21.1,11.97 21.6,12.47 23,12.47 | C16.+ 21.8,3.87 21.8,5.47 21,6.27 C15.2 21,6.47 21,7.47 v20.8,7.67 | v23,11.17 23,12.47 | U4.5 64.7,16.77 64.7,15.27 61.7,15.27 C14.2 61.6,15.37 61.6,18.27 v60.4,19.47 | v57.2,20.67 57.2,21.27 | 57.2,21.27 57.2,22.27 56.6,22.87 IC2.8 | v37.9,20.97 36.8,22.07 36.8,23.57 30.6,23.57 29.7,22.67 29.7,19.27 23,12.57 23,12.47 | v39.5,20.97 45.7,20.97 45.7,21.17 45.8,21.27 57.2,21.27
  top_internal 0.254: v57.2,20.67 58.4,19.47 v60.4,19.47 | v39.5,20.97 v37.9,20.97
  bottom_internal 0.254: v23,11.17 20.8,8.97 v20.8,7.67
+3V3  (via drill 0.61, 0.61 layers 1-2)
  Top 0.254: U9.8 29.9,7.67 31,7.67 U9.7 31.2,7.77 31.2,8.87 31.7,9.37 31.7,13.17 32.5,13.97 C32.2 37.5,13.87 39.8,11.57 v39.8,11.37 | 42,11.17 42,10.47 42.8,10.47 U6.18 | 42,11.17 42.2,11.37 42.8,11.37 U6.16 43,11.47 47.2,11.47 47.2,14.17 U6.6 47.3,14.27 47.3,14.97 48.7,16.37 48.8,16.37 | 48.8,16.17 48.8,14.27 U6.3 48.7,14.27 48.3,14.27 U6.4 | 48.8,16.17 48.8,16.37 | 48.8,16.37 48.8,17.67 C28.2 48.9,17.87 48.9,19.47 49.7,20.27 C27.+ | v40.9,12.47 42,11.37 42,11.17 | U12.8 90.2,1.97 91.5,1.97 91.5,12.47 90.7,13.27 90.2,13.27 U11.1 90,13.37 79.3,13.37 | 75.3,12.77 79.3,12.77 79.3,13.37 | 75.3,12.77 74.4,12.77 C33.2 | 79.3,13.37 79.3,15.17 C34.2 | v67.7,5.07 67.7,3.27 66.1,1.67 U7.5 | v75.3,12.67 75.3,12.77 | v55.7,16.17 48.8,16.17
  top_internal 0.254: v40.9,12.47 v39.8,11.37
  bottom_internal 0.254: v75.3,12.67 v67.7,5.07
  Bottom 0.254: v55.7,16.17 66.8,5.07 v67.7,5.07
+3V3_ISOL
  Top 0.254: 109.9,19.07 109.9,20.27 C35.1 | 109.9,19.07 109.9,17.87 C36.1 109.8,17.67 109,16.87 109,8.07 106.6,5.67 106.6,5.57 | 109.9,19.07 116.1,19.07 C42.2 116.2,18.97 116.2,3.87 C41.2 | 106.6,5.57 107.1,5.07 107.1,2.87 105.1,2.87 U15.8 104.9,2.77 104.5,2.77 104.1,2.37 104.1,1.97 97.6,1.97 | 106.6,5.57 105.1,5.57 105.1,5.47 U15.4 | 97.6,1.97 95.4,1.97 U12.1 | C38.+ 105.6,20.27 104.7,20.27 102.3,17.87 R26.2 102.2,17.67 97.9,13.37 97.6,13.37 | 97.6,13.37 95.4,13.37 U11.8 | 97.6,13.37 97.6,1.97
+5V_ISOL  (via drill 0.61, 0.61 layers 1-2)
  Top 0.254: v111.1,21.57 112,21.57 U13.1 | v113.6,22.77 113.6,21.87 113.9,21.57 U13.3 | v105.7,22.77 105.7,24.07 C37.+
  top_internal 0.254: v113.6,22.77 112.4,21.57 v111.1,21.57
  bottom_internal 0.254: 105.7,21.57 97.8,21.57 97.8,22.77 U10.P$1 | 105.7,21.57 v111.1,21.57 | 105.7,21.57 v105.7,22.77
-2.0V_NEG  (via drill 0.61 layers 1-2)
  Top 0.254: v70.8,10.77 70.8,10.17 C4.1 | v67.3,11.57 66.1,11.57 66.1,11.67 IC1.5 65.9,11.77 61.6,11.77 | 61.6,11.77 61.6,12.67 R5.2 61.5,12.77 61.5,14.07 61,14.57 61,15.77 60.5,16.27 60.5,17.57 60.4,17.67 IC2.4 | 61.6,11.77 61.6,11.37 61,10.77 61,8.27 61.6,7.67 C6.2 61.5,7.57 59.2,5.27 v59.2,4.77 | U$1.13 19.6,8.67 20,8.67 U$1.14 20.2,8.67 20.5,8.67 U$1.15 20.7,8.67 21,8.67 U$1.16 21.1,8.57 21.4,8.27 21.4,8.17 22.9,8.17 | 22.9,8.17 26.5,8.17 26.7,8.37 26.7,10.27 29.1,12.67 29.1,14.07 30.1,15.07 30.1,21.77 31.1,22.77 C7.2 | 22.9,8.17 22.9,2.27 21.9,1.27 C5.- 21.9,1.17 21.9,1.07 38.5,1.07 39.4,1.97 39.4,3.47 48.3,3.47 49,4.17 v49.9,4.17
  top_internal 0.254: v70.8,10.77 70,11.57 v67.3,11.57 | v59.2,4.77 58.9,4.47 50.2,4.47 v49.9,4.17
AGND  (via drill 0.61)  (1 unrouted)
  Top 0.254: 14,-54.63 14,-53.43 X4.2 14,-53.23 14,-31.83 X3.1 14,-31.73 14,-30.43 | 14,-54.63 14,-55.83 X4.1 | 19.1,-54.63 19.1,-53.43 X4.6 | 19.1,-54.63 19.1,-55.83 X4.5 | 19.1,-54.63 14,-54.63 | 14,-30.43 14,-29.23 X3.2 | 19.1,-30.43 19.1,-29.23 X3.6 | 19.1,-30.43 19.1,-31.73 X3.5 | 19.1,-30.43 14,-30.43 | 14,-29.13 X3.2 | 14,-29.03 X3.2 | 14,-28.93 X3.2 | 14,-6.33 14,-5.13 X2.2 | 14,-6.33 14,-7.53 X2.1 14,-7.73 14,-28.83 X3.2 | 19.1,-6.33 19.1,-5.13 X2.6 | 19.1,-6.33 19.1,-7.53 X2.5 | 19.1,-6.33 14,-6.33 | R28.2 73.1,1.27 v74.2,2.37 74.3,2.47 74.3,3.77 R17..2 74.2,3.87 73.7,4.37 73.7,10.67 73.75,10.72 | 73.75,10.72 73.7,10.77 73.7,14.57 74.3,15.17 R4.2 | 73.75,10.72 C4.2 | 60.3,8.47 60.3,10.07 C13.2 | 60.3,8.47 60.3,7.67 C6.1 | 60.3,8.47 v58.7,8.47 58.7,17.37 59,17.67 IC2.3 | 50.45,13.52 51,12.97 U6.48 51.1,12.87 51.1,12.47 U6.47 51,12.37 50.2,12.37 50.2,9.37 | 50.45,13.52 49.8,14.17 U6.1 | U6.42 51.1,9.87 51.1,9.47 U6.41 51,9.37 50.2,9.37 | 50.2,7.67 50.2,6.47 49.8,6.07 U6.36 | 50.2,7.67 50.4,7.87 51,7.87 U6.38 | 50.2,7.67 50.2,9.37 | U4.2 67.3,17.77 66.5,17.77 v66.5,15.97 66.5,14.37 67.7,13.17 67.7,12.37 68.3,11.77 68.6,11.77 IC1.1 | C15.1 19.6,6.27 18.9,5.57 v18.9,5.17 18.9,3.87 C16.- 18.9,3.77 18.9,1.27 C5.+ | C18.- 46,2.57 v47.7,2.57 49.3,2.57 C20.- | C7.1 v32.4,20.97 C43.1 | 79.4,10.17 79.4,11.37 C19.2 | 79.4,10.17 79.4,8.97 C17.2 | C22.1 55.2,7.67 v55.2,8.87 55.2,10.07 C23.1 | v23.7,6.37 24.7,6.37 C12.1 | v24.8,10.37 24.8,11.37 C11.1 | v56.5,13.77 56.5,12.77 C21.2 | v60.3,14.17 60.3,15.17 C14.1 | v67.4,7.67 68.6,7.67 U5.2 | v79.6,10.17 79.4,10.17 | v50.5,13.67 50.5,13.57 50.45,13.52
  pour Bottom: -1.27,26.67 91.44,26.67 91.44,0 0,0
  pour bottom_internal: -5.08,30.48 91.44,30.48 91.44,-2.54 -5.08,-2.54
GNDI  (15 unrouted)
  Top 0.254: 42.9,12.47 U6.14 42.9,12.47
  pour Top: -2.54,27.94 91.44,27.94 91.44,0 -2.54,0
  pour top_internal: -3.81,29.21 91.44,29.21 91.44,-1.27 -3.81,-1.27
ISOL_GND  (via drill 0.61)
  Top 0.254: 113.5,10.47 113.5,13.47 112.4,14.57 111.9,14.57 U14.4 | 113.5,10.47 113.5,5.27 114.9,3.87 C41.1 | 104.75,6.42 105,6.67 U15.2 105.1,6.77 105.1,7.27 U15.1 105,7.37 105,9.97 | 104.75,6.42 104.1,5.77 104.1,4.17 105,4.17 U15.6 | U15.3 105,6.07 104.8,6.27 104.8,6.37 104.75,6.42 | 105,9.97 102.3,12.67 R25.2 | U12.4 95.4,5.77 95.4,9.47 U11.5 95.2,9.57 92.8,9.57 92.8,18.67 95.3,21.17 95.3,21.27 | 102.7,21.27 102.7,24.07 C37.- | 102.7,21.27 102.7,20.37 C38.- | v112.1,3.47 110.9,3.47 U15.10 | 116.7,20.07 116.7,19.77 117.4,19.07 C42.1 | 116.7,20.07 116.7,20.67 | 116.7,20.67 116.7,23.57 116.2,24.07 C39.1 | 116.7,20.67 113.6,20.67 113.4,20.87 113.4,21.17 113.1,21.47 U13.2 113,21.67 113,21.87 112.4,22.47 111.3,22.47 109.8,23.97 C40.1 109.8,24.07 108.8,23.07 108.8,20.57 108.6,20.37 C35.2 108.6,20.27 108.6,17.87 C36.2 108.5,17.67 108.5,9.97 105,9.97 | v116.8,20.07 116.7,20.07 | 95.3,21.27 102.7,21.27 | 95.3,21.27 95.3,22.77 U10.P$2 | v113.6,10.47 113.5,10.47
  pour Bottom: 93.98,26.67 220.98,26.67 220.98,0 93.98,0
N$1
  Top 0.254: R6.2 4.4,1.27 3.2,2.47 3.2,3.77 C3.1 3.2,3.87 3.2,5.47 5.3,7.57 L1.2
N$2
  Top 0.254: R2.1 3.2,15.17 3.2,11.47 C1.1 3.1,11.37 3.1,8.37 2.4,7.67 L1.1
N$3
  Top 0.254: C3.2 4.5,3.77 9.5,3.77 R7.2 9.6,3.87 9.6,5.57 11.6,7.57 L2.2
N$4
  Top 0.254: C1.2 4.5,11.47 8.2,11.47 R3.1 8.3,11.37 8.3,7.97 8.6,7.67 L2.1
N$5
  Top 0.254: 14.6,0.57 16.4,0.57 16.5,0.67 16.5,9.87 18.8,9.87 U$1.11 | 14.6,0.57 R9.1 14.6,1.37 14.6,3.77 R11.2 14.6,3.87 14.6,7.57 C9.1 | 14.6,0.57 3.9,0.57 3.2,1.27 R6.1
N$6  (via drill 0.61, 0.61 layers 1-2)
  Top 0.254: R8.1 10.8,3.77 R7.1 10.9,3.87 v13.7,6.67 | 23.8,9.87 24.2,9.87 24.2,9.47 24.7,8.97 R12.2 | 23.8,9.87 21.8,9.87 U$1.2 | v31.9,14.47 31.9,15.97 32.4,16.47 C10.1 | 23.8,9.87 v23.8,9.57
  top_internal 0.254: v13.7,6.67 16.6,9.57 v23.8,9.57
  bottom_internal 0.254: v31.9,14.47 27,9.57 v23.8,9.57
N$7
  Top 0.254: R20.2 24.8,2.47 25.5,1.77 29.8,1.77 29.8,2.47 U9.1
N$8
  Top 0.254: X1.3 16.5,16.47 14.8,14.77 14.8,12.87 13.4,11.47 R1.2 13.3,11.37 13.3,10.67 9.1,10.67 8.9,10.87 8.9,12.17 7.5,12.17 4.5,15.17 R2.2
N$9
  Top 0.254: R3.2 9.6,11.47 12,11.47 R1.1 12,11.57 14.4,13.97 14.4,15.47 15.5,16.57 15.5,17.97 16.5,18.97 X1.4
N$10
  Top 0.254: R11.1 15.9,3.87 15.9,7.57 C9.2 15.9,7.67 15.9,10.47 | 15.9,10.47 18.8,10.47 U$1.10 | 15.9,10.47 15.9,11.37 R14.2
N$11  (via drill 0.61 layers 1-2)
  Top 0.254: C10.2 31.1,13.57 | 31.1,13.57 R15.2 | 26.7,13.27 25,13.27 24,12.27 24,10.37 21.8,10.37 U$1.3 | 26.7,13.27 26.7,10.87 26.1,10.27 26.1,8.97 R12.1 | v30.3,13.57 31.1,13.57 | v28.3,13.47 26.7,13.47 26.7,13.27
  top_internal 0.254: v30.3,13.57 30.2,13.47 v28.3,13.47
N$12  (via drill 0.61 layers 1-2)
  Top 0.254: R14.1 18,12.27 v18,12.47 | v25.3,12.47 26,11.77 26,11.47 C11.2 | v52.3,8.37 51.1,8.37 U6.39
  top_internal 0.254: v18,12.47 v25.3,12.47 26.1,12.47 28.8,9.77 50.9,9.77 v52.3,8.37
N$13  (via drill 0.61)
  Top 0.254: R15.1 32.4,11.37 | 32.4,11.37 32.4,9.47 31.8,8.87 31.8,6.27 26.1,6.27 C12.2 | v52.3,9.57 52.3,10.37 51.1,10.37 U6.43 | 32.4,11.37 v38.6,11.37
  bottom_internal 0.254: v52.3,9.57 50.5,11.37 v38.6,11.37
N$16  (via drill 0.61 layers 1-2)
  Top 0.254: X1.9 24.1,16.57 24.1,18.97 X1.10 | U10.P$7 82.5,22.77 79.8,20.07 73.4,20.07 73.4,19.17 C2..- 73.4,18.97 72.2,17.77 72.2,13.67 69.6,13.67 69.5,13.57 68.8,13.57 IC1.3 68.7,13.57 68.7,12.77 IC1.2 68.8,12.77 69.5,12.07 69.5,10.77 v62.6,10.77
  top_internal 0.254: v62.6,10.77 58.4,10.77 53.9,15.27 25.4,15.27 24.2,16.47 X1.9
N$17  (via drill 0.61 layers 1-2)
  Top 0.254: v74.9,11.57 74.9,8.67 77.4,8.67 77.6,8.87 78,8.87 C17.1 | v66.8,19.67 64.8,19.67 64.8,18.77 U4.4
  top_internal 0.254: v66.8,19.67 v74.9,11.57
N$18  (via drill 0.61 layers 1-2)
  Top 0.254: X1.7 21.6,16.57 21.6,18.97 X1.8 21.7,19.07 26.6,23.97 v48.5,23.97 | U7.1 68.7,1.67 69.5,1.67 69.5,2.87 68.9,3.47 68.7,3.47 U7.3 68.7,3.57 68.7,6.67 U5.1 68.8,6.57 69.5,7.27 69.5,8.57 | 69.5,8.57 U5.3 | 68.2,16.87 67.4,16.87 U4.1 | 68.2,16.87 68.2,18.17 67.7,18.67 67.4,18.67 U4.3 67.7,18.77 67.7,21.17 | 67.7,21.17 67.7,21.57 67.4,21.87 U8.1 67.6,21.77 68.2,22.37 68.2,22.87 | 68.2,22.87 68.2,23.77 67.4,23.77 U8.3 | 68.2,22.87 73.4,22.87 C25.+ 73.5,22.97 73.5,24.47 83.4,24.47 85,22.87 U10.P$6 | v69.9,12.87 69.9,9.07 69.5,8.67 69.5,8.57 | v69.9,14.47 68.2,16.17 68.2,16.87 | 67.7,21.17 v60.4,21.17
  top_internal 0.254: v69.9,14.47 v69.9,12.87 | v48.5,23.97 51,21.47 60.1,21.47 v60.4,21.17
N$20  (via drill 0.61 layers 1-2)
  Top 0.254: v77.1,9.47 77.1,10.47 78,11.37 C19.1 | v67.6,9.37 66.1,9.37 66.1,8.57 U5.4
  top_internal 0.254: v77.1,9.47 77,9.37 v67.6,9.37
N$22
  Top 0.254: X4.9 24.1,-55.83 24.1,-53.43 X4.10 24.2,-53.23 24.2,-31.83 X3.9 24.1,-31.73 24.1,-29.23 X3.10 | 24.2,-29.13 X3.10 | 24.2,-29.03 X3.10 | 24.2,-28.93 X3.10 | X2.10 24.1,-5.13 24.1,-7.53 X2.9 24.2,-7.73 24.2,-28.83 X3.10
N$23
  Top 0.254: C31.1 49,22.87 49.3,23.17 49.3,24.47 49.5,24.67 64.7,24.67 64.7,23.87 U8.4
N$24
  Top 0.254: X4.7 21.6,-55.83 21.6,-53.43 X4.8 21.6,-53.23 21.6,-31.83 X3.7 21.6,-31.73 21.6,-29.23 X3.8 | 21.6,-29.13 X3.8 | 21.6,-29.03 X3.8 | 21.6,-28.93 X3.8 | X2.8 21.6,-5.13 21.6,-7.53 X2.7 21.6,-7.73 21.6,-28.83 X3.8
N$26
  Top 0.254: C26.1 73,7.57 69.9,4.47 69.9,1.47 69.5,1.07 65.1,1.07 65.1,2.57 66,3.47 U7.4
N$27  (via drill 0.61 layers 1-2)
  Top 0.254: v60.7,11.57 60.7,12.37 60.4,12.67 R5.1 | v62.6,12.57 66,12.57 66,13.57 IC1.4 | v70.7,11.97 71.1,11.97 72.6,13.47 72.6,14.77 73,15.17 R4.1
  top_internal 0.254: v60.7,11.57 61.7,12.57 v62.6,12.57 67.4,12.57 67.9,12.07 70.6,12.07 v70.7,11.97
N$28  (via drill 0.61 layers 1-2)
  Top 0.254: IC2.6 59,22.97 57.8,22.97 IC2.7 58,22.87 58,20.37 57.1,19.47 50.8,19.47 v50.3,18.97 | v18.8,11.67 18.8,10.97 U$1.9 | v21.9,11.67 21.8,11.57 21.8,10.97 U$1.4 | 30.55,18.42 30.5,18.37 30.5,14.87 29.5,13.87 29.5,11.97 v27.5,9.97 | 30.55,18.42 31.1,18.97 C43.2 | v37.9,18.87 33,18.87 33,18.47 32.9,18.37 30.6,18.37 30.55,18.42
  top_internal 0.254: v18.8,11.67 v21.9,11.67 22,11.67 22.3,11.97 23.3,11.97 23.6,11.67 25.8,11.67 v27.5,9.97 | v50.3,18.97 50.2,18.87 v37.9,18.87
N$30  (via drill 0.61 layers 1-2)
  Top 0.254: v56.6,1.47 56.6,2.47 R16.2 | v58.2,1.47 61.6,1.47 61.6,2.47 R13.1 61.7,2.57 61.7,2.97 62.2,3.47 62.2,9.07 | C13.1 62.2,9.57 62.2,9.07 | v59.5,9.27 59.5,14.47 59.6,14.57 59.6,22.17 60.3,22.87 IC2.5 | 62.2,9.07 v61.8,9.07
  top_internal 0.254: v58.2,1.47 v56.6,1.47 | v59.5,9.27 59.7,9.07 v61.8,9.07
N$31  (via drill 0.61 layers 1-2)
  Top 0.254: v33,5.57 29.1,5.57 26.1,2.57 R20.1 | v34.6,7.17 37,9.57 42,9.57 42,8.67 42.2,8.47 42.8,8.47 U6.22
  top_internal 0.254: v34.6,7.17 v33,5.57
N$32
  Top 0.254: R16.1 55.2,2.57 52.3,2.57 C20.+ 52.3,6.17 51.1,7.37 U6.37
N$33
  Top 0.254: C21.1 55.2,12.67 52,12.67 52,12.17 51.8,11.97 51.1,11.97 U6.46
N$34  (via drill 0.61 layers 1-2)
  Top 0.254: v109.6,4.07 110.8,4.07 U15.11
  top_internal 0.254: v109.6,4.07 110.3,4.77 122.9,4.77 124.4,6.27 X5.1
N$35  (via drill 0.61 layers 1-2)
  Top 0.254: v112.3,5.57 112.3,4.77 110.9,4.77 U15.12
  top_internal 0.254: v112.3,5.57 113,6.27 121.9,6.27 X5.2
N$36
  Top 0.254: R19.1 38.8,8.87 39.7,7.97 42.8,7.97 U6.23
N$37
  Top 0.254: 36.8,6.27 36.8,8.27 37.4,8.87 R19.2 | 36.8,6.27 36.8,3.17 37.4,2.57 R18.2 | 36.8,6.27 33.3,6.27 33.1,6.47 33.1,6.97 32.4,7.67 U9.6
N$38
  Top 0.254: R18.1 38.8,2.57 39,2.77 39,3.67 40.5,5.17 46.2,5.17 46.2,5.97 U6.29
N$39
  Top 0.254: U9.2 31.2,2.57 32.3,2.57 U9.3
N$40  (via drill 0.61 layers 1-2)
  Top 0.254: R10.2 56.5,17.67 IC2.1 56.4,17.07 52.2,17.07 51.5,17.77 C8.1 51.3,17.77 v49.9,17.77 | 15.2,9.57 15.3,9.57 15.3,1.77 15.8,1.27 R9.2 | 15.2,9.57 14.2,9.57 13.6,8.97 13.6,7.77 10.2,4.37 10.2,1.87 9.6,1.27 R8.2 | v27.3,18.07 22.5,13.27 15.2,13.27 15.2,9.57
  top_internal 0.254: v49.9,17.77 49.6,18.07 v27.3,18.07
N$41
  Top 0.254: C8.2 52.8,17.87 55.9,17.87 55.9,18.87 56.1,19.07 57.7,19.07 57.7,17.77 IC2.2 57.8,17.67 R10.1 57.8,5.07 60.3,2.57 R13.2
N$42  (via drill 0.61 layers 1-2)
  Top 0.254: v40.6,10.57 36.5,10.57 33.7,7.77 U9.5 | v75.3,7.87 78.8,7.87 78.8,11.97 79,12.17 90.1,12.17 U11.2
  top_internal 0.254: v40.6,10.57 40.8,10.37 61.9,10.37 63.8,8.47 74.7,8.47 v75.3,7.87
N$43
  Top 0.254: R21.1 38.8,5.17 39.9,5.17 41.7,6.97 43.8,6.97 43.8,8.67 43.6,8.87 42.9,8.87 U6.21
N$44  (via drill 0.61 layers 1-2)
  Top 0.254: v38,6.17 38,5.67 37.5,5.17 R21.2 | v74.5,6.17 78.5,6.17 80.6,8.27 88.7,8.27 88.7,9.87 89.6,10.77 90.1,10.77 U11.3
  top_internal 0.254: v74.5,6.17 v38,6.17
N$45  (via drill 0.61 layers 1-2)
  Top 0.254: 55.9,3.67 55.9,2.07 55.4,1.57 50.7,1.57 50.7,4.47 50,5.17 49.3,5.17 49.3,5.97 U6.35 | 55.9,3.67 55.9,4.47 56.5,5.07 C24.2 | v75.3,4.37 78.6,4.37 79.3,5.07 R17.2 | 55.9,3.67 v56.6,3.67
  top_internal 0.254: v75.3,4.37 74.6,3.67 v56.6,3.67
N$46
  Top 0.254: R17.1 78.1,5.17 78.8,5.87 88.7,5.87 88.7,5.37 89.6,4.47 90.1,4.47 U12.6
N$47  (via drill 0.61 layers 1-2)
  Top 0.254: v48.3,4.57 48.7,4.97 48.7,5.97 U6.34 | v63,2.57 65,0.57 88.7,0.57 88.7,2.27 89.6,3.17 U12.7
  top_internal 0.254: v48.3,4.57 50.3,2.57 v63,2.57
N$50
  Top 0.254: 113.1,4.37 116.2,1.27 R27.1 | 113.1,4.37 113.1,9.57 111.9,10.77 U14.1 | U12.3 95.3,4.37 93.9,4.37 93.9,1.57 94.4,1.07 113,1.07 113,4.37 113.1,4.37
N$51  (via drill 0.61 layers 1-2)
  Top 0.254: v103.8,7.27 103.8,8.67 99.8,12.67 R24.2 | v106.3,4.77 105.1,4.77 U15.5
  top_internal 0.254: v106.3,4.77 v103.8,7.27
N$52
  Top 0.254: R23.2 103.7,6.17 103.7,3.97 104.2,3.47 105,3.47 U15.7
N$53  (via drill 0.61 layers 1-2)
  Top 0.254: v98.4,11.57 98.4,12.67 R24.1 | v93.6,11.57 95.3,11.57 95.3,11.97 U11.7
  top_internal 0.254: v93.6,11.57 v98.4,11.57
N$54  (via drill 0.61 layers 1-2)
  Top 0.254: v98.4,9.07 98.4,10.07 R23.1 | v96.8,8.67 96.7,8.77 96.7,9.87 95.8,10.77 95.4,10.77 U11.6
  top_internal 0.254: v98.4,9.07 98,8.67 v96.8,8.67
N$55  (via drill 0.61 layers 1-2)
  Top 0.254: v109.6,5.27 109.6,5.37 110.8,5.37 U15.13
  top_internal 0.254: v109.6,5.27 112.2,7.87 123.4,7.87 124.4,8.87 X5.3
N$56  (via drill 0.61 layers 1-2)
  Top 0.254: v113.8,1.27 R27.2 | v112.1,2.07 111.4,2.77 110.9,2.77 U15.9
  top_internal 0.254: v113.8,1.27 113,2.07 v112.1,2.07
N$57  (via drill 0.61 layers 1-2)
  Top 0.254: v107.1,17.77 103.6,17.77 R26.1 | v96.8,6.57 96.8,3.27 95.4,3.27 U12.2
  top_internal 0.254: 107.65,17.22 110.9,13.97 X5.8 | 107.65,17.22 v107.1,17.77 | v96.8,6.57 98.5,8.27 98.7,8.27 107.65,17.22
N$58  (via drill 0.61 layers 1-2)
  Top 0.254: v109.3,6.47 109.3,6.07 110.8,6.07 U15.14
  top_internal 0.254: v109.3,6.47 111.7,8.87 121.9,8.87 X5.4
N$59
  Top 0.254: U14.2 111.9,12.07 111.9,13.27 U14.3
N$60  (via drill 0.61)
  Top 0.254: 104.9,12.77 106.6,12.77 106.6,13.27 U14.6 | 104.9,12.77 103.6,12.77 R25.1 | v104.9,12.87 104.9,12.77
  bottom_internal 0.254: v104.9,12.87 124.4,12.87 124.4,13.97 X5.7
N$61  (via drill 0.61 layers 1-2)
  Top 0.254: v100.3,14.67 106.6,14.67 U14.5
  top_internal 0.254: v100.3,14.67 99.8,15.17 97.8,15.17 U10.P$14
N$62  (via drill 0.61 layers 1-2)
  Top 0.254: 107.9,23.07 107.9,15.07 108,14.97 108,12.17 107.25,11.42 | 107.9,23.07 107.9,23.47 108.5,24.07 C40.2 | 107.25,11.42 106.7,10.87 U14.8 | v110.9,24.07 112,24.07 U13.5 | v108,23.07 107.9,23.07 | 107.25,11.42 106.7,11.97 U14.7
  top_internal 0.254: v110.9,24.07 109.9,23.07 v108,23.07
N$63  (via drill 0.61 layers 1-2)
  Top 0.254: v110,9.67 110,6.77 110.8,6.77 U15.15
  top_internal 0.254: v110,9.67 112.8,12.47 123.4,12.47 124.4,11.47 X5.5
N$64  (via drill 0.61 layers 1-2)
  Top 0.254: v117.5,23.07 117.5,24.07 C39.2 | v114.8,23.27 114,24.07 U13.4
  top_internal 0.254: v117.5,23.07 117.3,23.27 v114.8,23.27
N$65  (via drill 0.61)
  Top 0.254: v112.3,6.87 112.3,7.27 110.9,7.27 U15.16
  bottom_internal 0.254: v112.3,6.87 116.8,11.37 121.9,11.37 X5.6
